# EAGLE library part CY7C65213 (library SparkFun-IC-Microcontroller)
CY7C65213 USB-UART controller USB UART SparkFun Products None
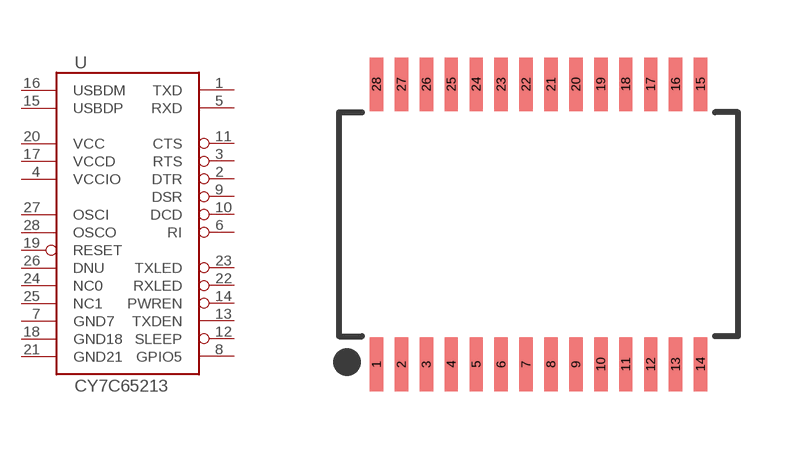
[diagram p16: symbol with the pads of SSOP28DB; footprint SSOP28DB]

Designator prefix U

## CY7C65213 (PROD_ID: IC-12487)  [SSOP28DB]
1  TXD  out
2  DTR  out
3  RTS  out
4  VCCIO  pwr
5  RXD  in
6  RI  in
7  GND7  pwr
8  GPIO5  in
9  DSR  in
10  DCD  in
11  CTS  in
12  SLEEP  in
13  TXDEN  in
14  PWREN  in
15  USBDP
16  USBDM
17  VCCD  out
18  GND18  pwr
19  RESET  in
20  VCC  pwr
21  GND21  pwr
22  RXLED  in
23  TXLED  in
24  NC0  in
25  NC1  pwr
26  DNU  in
27  OSCI  in
28  OSCO  out

## Footprint SSOP28DB (pad centres in mm)
Small Shrink Outline Package
smd 0.348 x 1.397: 1 -4.225,-3.656; 2 -3.575,-3.656; 3 -2.925,-3.656; 4 -2.275,-3.656; 5 -1.625,-3.656; 6 -0.975,-3.656; 7 -0.325,-3.656; 8 0.325,-3.656; 9 0.975,-3.656; 10 1.625,-3.656; 11 2.275,-3.656; 12 2.925,-3.656; 13 3.575,-3.656; 14 4.225,-3.656; 15 4.225,3.656; 16 3.575,3.656; 17 2.925,3.656; 18 2.275,3.656; 19 1.625,3.656; 20 0.975,3.656; 21 0.325,3.656; 22 -0.325,3.656; 23 -0.975,3.656; 24 -1.625,3.656; 25 -2.275,3.656; 26 -2.925,3.656; 27 -3.575,3.656; 28 -4.225,3.656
